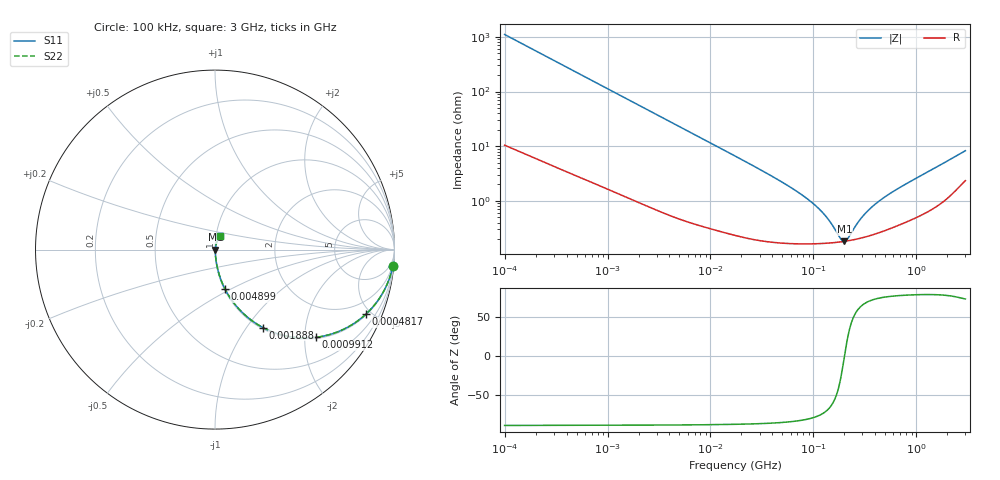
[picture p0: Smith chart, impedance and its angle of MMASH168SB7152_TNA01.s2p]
! MMASH168SB7152_TNA01  S-PARAMETER MODEL  ( Standard Model )
! Model Generated by TAIYO YUDEN Corporation (http://www.ty-top.com)
! Version 1.0
! TAIYO YUDEN Control No. 220601
! Copyright(c) 2013 TAIYO YUDEN CO.,LTD. All Rights Reserved.
! Product Description (link to TY-COMPAS)
! https://ds.yuden.co.jp/TYCOMPAS/or/detail?pn=MMASH168SB7152KTNA01&u=M
! Products Name : Multilayer Ceramic Capacitors
! Characteristics :
!  Capacitance : 1500 [pF] , Rated Voltage : 100 [V] , TCC : X7R
!  Case Size : 1.6 x 0.8 / 0.063 x 0.031 [mm/inch] , Thickness : 0.8 / 0.031 [mm/inch]
!  (Conditions: Temperature = 25 [degC] , DC Bias Voltage = 0 [V])
! External Node Assignments :
!  1  o---| |---o  2
! GND o---------o GND
! Frequency Range : 100kHz  -  3GHz  [ 401 STEP ]
# MHZ S RI R 50
! Freq[MHz].  S11 Real  S11 Imag  S21 Real  S21 Imag  S12 Real  S12 Imag  S22 Real  S22 Imag
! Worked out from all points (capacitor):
!   401 points, 100 kHz to 3 GHz, reference 50 ohm
!   read as one part in series: C = 1.43 nF near 105.3 kHz
!   lowest |Z| = 182 mohm at 200.4 MHz (marker M1)
!   series resonance near 200.6 MHz, so ESL is about 440 pH
!   S11 on the Smith chart (normalised r, x): 100 kHz: 1, -22; 481.7 kHz: 1.06, -4.65; 991.2 kHz: 1.03, -2.27; 1.888 MHz: 1.02, -1.20; 4.899 MHz: 1.01, -0.47; 3 GHz: 1.05, +0.16
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0.1  0.9911 -0.0894  0.00891 0.0894  0.00891 0.0894  0.9911 -0.0894
0.252895  0.9489 -0.2147  0.0511 0.2147  0.0511 0.2147  0.9489 -0.2147
0.481683  0.8407 -0.3596  0.1593 0.3596  0.1593 0.3596  0.8407 -0.3596
0.562235  0.796 -0.3965  0.204 0.3965  0.204 0.3965  0.796 -0.3965
0.991196  0.5628 -0.4888  0.4372 0.4888  0.4372 0.4888  0.5628 -0.4888
1.350433  0.413 -0.4848  0.587 0.4848  0.587 0.4848  0.413 -0.4848
1.887902  0.2682 -0.435  0.7318 0.435  0.7318 0.435  0.2682 -0.435
3.161081  0.1192 -0.3152  0.8808 0.3152  0.8808 0.3152  0.1192 -0.3152
4.899066  0.0556 -0.2192  0.9444 0.2192  0.9444 0.2192  0.0556 -0.2192
8.862326  0.0196 -0.1265  0.9804 0.1265  0.9804 0.1265  0.0196 -0.1265
17.7727  0.00644 -0.0641  0.9936 0.0641  0.9936 0.0641  0.00644 -0.0641
52.46276  0.0021 -0.0206  0.9979 0.0206  0.9979 0.0206  0.0021 -0.0206
97.38194  0.00172 -0.0091  0.9983 0.0091  0.9983 0.0091  0.00172 -0.0091
129.3002  0.0017 -0.00523  0.9983 0.00523  0.9983 0.00523  0.0017 -0.00523
180.7614  0.00177 -0.0012  0.9982 0.0012  0.9982 0.0012  0.00177 -0.0012
200.3904  0.00182 -1.25e-05  0.9982 1.25e-05  0.9982 1.25e-05  0.00182 -1.25e-05
216.4987  0.00186 0.000874  0.9981 -0.000874  0.9981 -0.000874  0.00186 0.000874
273.0175  0.00204 0.00356  0.998 -0.00356  0.998 -0.00356  0.00204 0.00356
326.9943  0.00224 0.00575  0.9978 -0.00575  0.9978 -0.00575  0.00224 0.00575
412.3589  0.0026 0.00877  0.9974 -0.00877  0.9974 -0.00877  0.0026 0.00877
547.5153  0.00323 0.013  0.9968 -0.013  0.9968 -0.013  0.00323 0.013
3000  0.0288 0.0753  0.9712 -0.0753  0.9712 -0.0753  0.0288 0.0753
